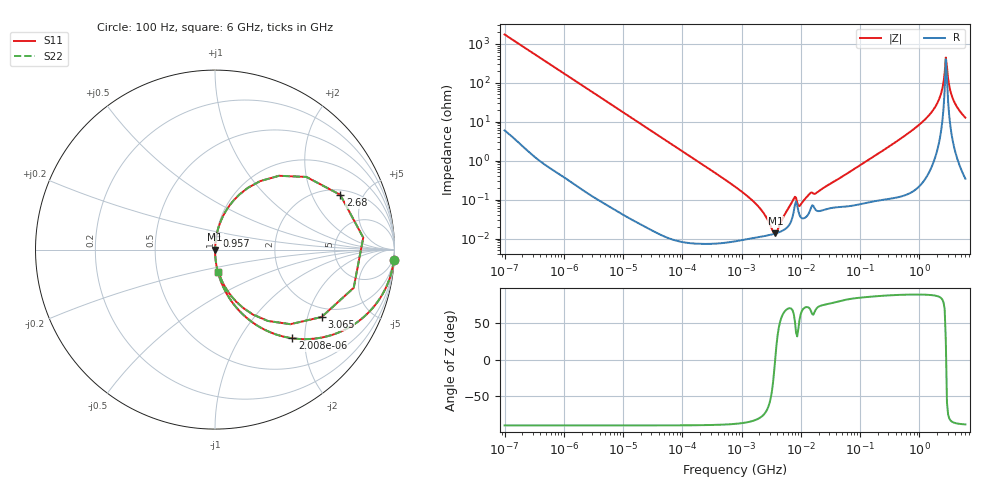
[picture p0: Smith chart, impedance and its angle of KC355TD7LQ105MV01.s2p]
!Murata Part Number: KC355TD7LQ105MV01
!These Parameters are Measured in Series Mode Connection
!Data Generated on Mar 13, 2026
!  o--ll--o
!Port1  Port2
!  o------o
!Operation Temp=25[degC], DC Bias Voltage=0[V]
!Freq. Start=100[Hz] Stop=6[GHz] 401[Steps]
# Hz S RI R 50
!Freq.(Hz) S11(Real) S11(Imag) S21(Real) S21(Imag) S12(Real) S12(Imag) S22(Real) S22(Imag)
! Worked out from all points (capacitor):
!   401 points, 100 Hz to 6 GHz, reference 50 ohm
!   read as one part in series: C = 915 nF near 109 Hz
!   lowest |Z| = 13.4 mohm at 3.712 MHz (marker M1)
!   series resonance near 3.691 MHz, so ESL is about 2 nH
!   S11 on the Smith chart (normalised r, x): 100 Hz: 1, -35; 2.008 kHz: 1.00, -1.74; 957 MHz: 1.00, +0.16; 2.68 GHz: 2.28, +3.31; 3.065 GHz: 1.66, -2.46; 6 GHz: 1.01, -0.25
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100  0.9965 -0.0574  0.0035 0.0574  0.0035 0.0574  0.9965 -0.0574
600  0.8935 -0.3074  0.1065 0.3074  0.1065 0.3074  0.8935 -0.3074
2008  0.4302 -0.4941  0.5698 0.4941  0.5698 0.4941  0.4302 -0.4941
6151  0.0751 -0.2625  0.9249 0.2625  0.9249 0.2625  0.0751 -0.2625
40335  0.00201 -0.0433  0.998 0.0433  0.998 0.0433  0.00201 -0.0433
774597  8.91e-05 -0.00215  0.9999 0.00215  0.9999 0.00215  8.91e-05 -0.00215
1896632  0.000108 -0.000671  0.9999 0.000671  0.9999 0.000671  0.000108 -0.000671
3712478  0.000134 5.7e-06  0.9999 -5.7e-06  0.9999 -5.7e-06  0.000134 5.7e-06
7599586  0.000496 0.000936  0.9995 -0.000936  0.9995 -0.000936  0.000496 0.000936
9941735  0.000354 0.000653  0.9996 -0.000653  0.9996 -0.000653  0.000354 0.000653
1.555665e7  0.000714 0.00133  0.9993 -0.00133  0.9993 -0.00133  0.000714 0.00133
3.124326e8  0.00158 0.0233  0.9984 -0.0233  0.9984 -0.0233  0.00158 0.0233
9.569533e8  0.00827 0.0785  0.9917 -0.0785  0.9917 -0.0785  0.00827 0.0785
1.497423e9  0.0278 0.1478  0.9722 -0.1478  0.9722 -0.1478  0.0278 0.1478
2.048624e9  0.1058 0.2764  0.8942 -0.2764  0.8942 -0.2764  0.1058 0.2764
2.450438e9  0.3564 0.4112  0.6436 -0.4112  0.6436 -0.4112  0.3564 0.4112
2.679998e9  0.6977 0.3053  0.3023 -0.3053  0.3023 -0.3053  0.6977 0.3053
2.802721e9  0.826 0.0669  0.174 -0.0669  0.174 -0.0669  0.826 0.0669
3.065283e9  0.594 -0.3755  0.406 0.3755  0.406 0.3755  0.594 -0.3755
3.352442e9  0.2946 -0.3976  0.7054 0.3976  0.7054 0.3976  0.2946 -0.3976
3.8344e9  0.119 -0.2909  0.881 0.2909  0.881 0.2909  0.119 -0.2909
6e9  0.0191 -0.1241  0.9809 0.1241  0.9809 0.1241  0.0191 -0.1241
